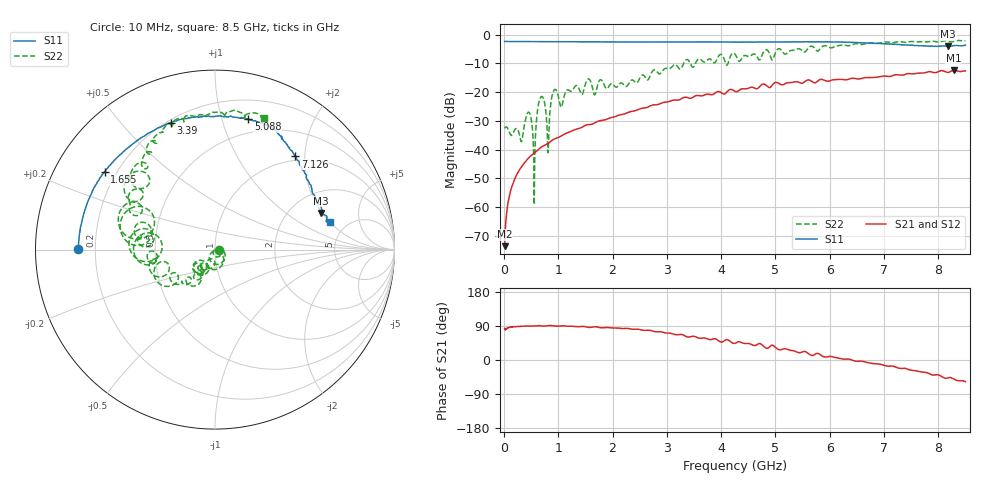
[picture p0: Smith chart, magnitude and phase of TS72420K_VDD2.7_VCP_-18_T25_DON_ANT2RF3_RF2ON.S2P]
!Agilent Technologies,E5071C,MY46417908,A.11.23
!Date: Thu Oct 03 16:41:04 2019
!Data & Calibration Information:
!Freq	S11:SOLT2(ON)	S21:SOLT2(ON)	S12:SOLT2(ON)	S22:SOLT2(ON)
!PortZ  Port1:50+j0  Port2:50+j0
!Above PortZ is port z conversion or system Z0 setting when saving the data.
!When reading, reference impedance value at option line is always used.
# Hz S dB R 50
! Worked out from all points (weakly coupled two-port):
!   1601 points, 10 MHz to 8.5 GHz, reference 50 ohm
!   highest |S21| = -12.43 dB at 8.288 GHz (marker M1); lowest = -73.6 dB at 10 MHz (marker M2)
!   lowest |S11| = -4.1 dB at 8.182 GHz (marker M3), VSWR 4.32, Z = 145 + j97.2 ohm
!   |S11| at or under -10 dB: nowhere
!   |S22| runs from -59.2 to -2.0 dB; largest |S21 - S12| = 0.0028
!   S11 on the Smith chart (normalised r, x): 10 MHz: 0.13, +0.00; 1.655 GHz: 0.16, +0.31; 3.39 GHz: 0.21, +0.69; 5.088 GHz: 0.37, +1.22; 7.126 GHz: 0.92, +1.81; 8.5 GHz: 3.66, +2.01
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1e7  -2.34 179.8  -73.61 83.2  -74.35 69.6  -32.57 0.1
1.108188e8  -2.37 177.3  -55.00 87.0  -54.99 86.8  -34.50 -24.4
3.230688e8  -2.39 172.4  -45.97 88.8  -45.95 89.0  -37.18 -19.2
4.55725e8  -2.40 169.5  -42.84 89.5  -42.86 89.5  -26.97 -61.4
5.6185e8  -2.41 167.1  -41.08 90.0  -41.09 89.8  -48.17 50.1
6.838938e8  -2.42 164.4  -39.14 89.9  -39.14 89.8  -21.56 -66.7
8.059375e8  -2.41 161.6  -37.88 90.5  -37.88 90.5  -39.92 -113.9
9.279812e8  -2.42 159.1  -36.28 89.8  -36.27 89.9  -19.16 -87.0
1.050025e9  -2.43 156.6  -35.30 90.0  -35.31 90.1  -25.25 -108.7
1.426769e9  -2.45 149.1  -32.30 88.6  -32.30 88.7  -20.79 -125.6
1.554119e9  -2.44 146.7  -31.29 86.2  -31.28 86.2  -15.38 -128.6
1.654938e9  -2.47 144.9  -30.89 87.6  -30.88 87.5  -20.56 -139.4
2.843538e9  -2.53 120.3  -24.27 74.5  -24.26 74.5  -13.46 -133.9
3.390081e9  -2.52 109.3  -21.96 60.5  -21.95 60.5  -8.77 -159.3
4.255e9  -2.57 92.3  -19.71 44.1  -19.69 44.0  -6.78 167.8
5.088081e9  -2.50 75.7  -17.24 26.7  -17.18 26.5  -5.01 154.0
5.671769e9  -2.48 67.1  -16.27 12.1  -16.23 12.5  -4.00 138.7
7.088538e9  -3.23 49.8  -14.56 -16.4  -14.50 -16.1  -2.59 109.2
7.125681e9  -3.28 49.2  -14.48 -15.9  -14.47 -15.8  -2.76 108.4
8.181625e9  -4.09 19.1  -13.15 -47.1  -13.19 -47.3  -2.28 78.0
8.28775e9  -3.78 17.1  -12.43 -50.4  -12.43 -50.7  -2.34 77.5
8.5e9  -3.65 13.8  -12.61 -57.1  -12.64 -57.3  -2.11 69.6
